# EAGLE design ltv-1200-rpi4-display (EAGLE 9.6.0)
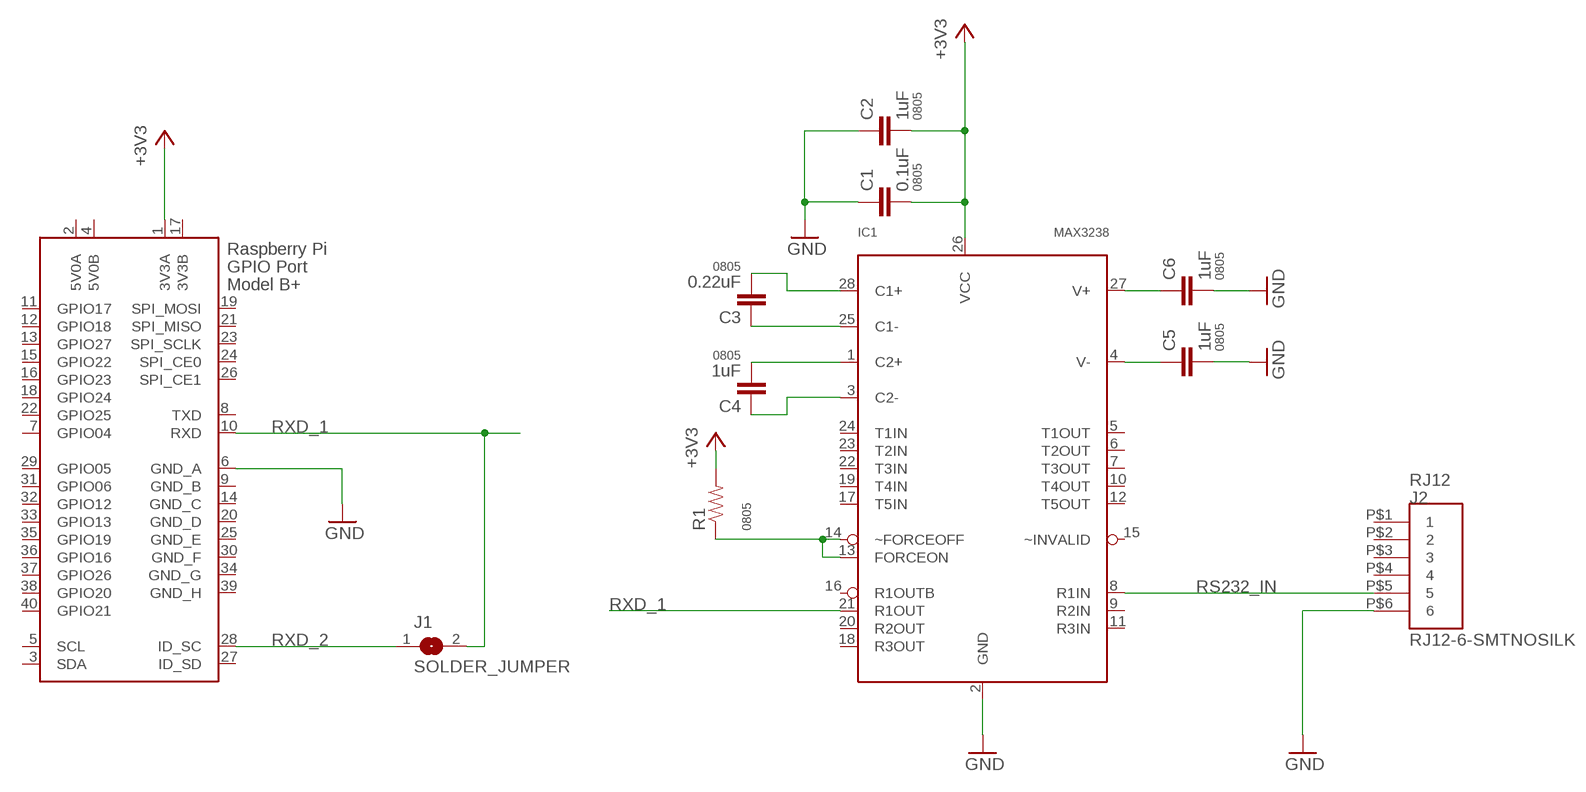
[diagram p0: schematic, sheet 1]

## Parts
C1  0.1uF  CAP0805  [0805]
C2  1uF  CAP0805  [0805]
C3  0.22uF  CAP0805  [0805]
C4  1uF  CAP0805  [0805]
C5  1uF  CAP0805  [0805]
C6  1uF  CAP0805  [0805]
IC1  MAX3238  [SSOP28]
J1  SOLDER_JUMPER  [SOLDER_JUMPER]
J2  RJ12-6-SMTNOSILK  [RJ12-6-SMT-NOSILK]
R1  RESISTOR0805-RES  [0805]
X1  RASPI_BOARD_B+#_F  [RASPI_BOARD_B+_FULL]

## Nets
+3V3: C1.2 C2.2 IC1.26(VCC) R1.2 X1.1(3V3A)
GND: C1.1 C2.1 C5.2 C6.2 IC1.2(GND) J2.P$6 X1.6(GND_A)
N$1: C3.2 IC1.28(C1+)
N$2: C3.1 IC1.25(C1-)
N$3: C4.2 IC1.1(C2+)
N$4: C4.1 IC1.3(C2-)
N$5: C6.1 IC1.27(V+)
N$6: C5.1 IC1.4(V-)
N$7: IC1.13(FORCEON) IC1.14(~FORCEOFF) R1.1
RS232_IN: IC1.8(R1IN) J2.P$5
RXD_1: IC1.21(R1OUT) J1.2 X1.10(RXD)
RXD_2: J1.1 X1.28(ID_SC)
Unconnected: IC1.5(T1OUT) IC1.6(T2OUT) IC1.7(T3OUT) IC1.9(R2IN) IC1.10(T4OUT) IC1.11(R3IN) IC1.12(T5OUT) IC1.15(~INVALID) IC1.16(R1OUTB) IC1.17(T5IN) IC1.18(R3OUT) IC1.19(T4IN) IC1.20(R2OUT) IC1.22(T3IN) IC1.23(T2IN) IC1.24(T1IN) J2.P$1 J2.P$2 J2.P$3 J2.P$4 X1.3(SDA) X1.5(SCL) X1.7(GPIO04) X1.8(TXD) X1.11(GPIO17) X1.12(GPIO18) X1.13(GPIO27) X1.15(GPIO22) X1.16(GPIO23) X1.18(GPIO24) X1.19(SPI_MOSI) X1.21(SPI_MISO) X1.22(GPIO25) X1.23(SPI_SCLK) X1.24(SPI_CE0) X1.26(SPI_CE1) X1.27(ID_SD) X1.29(GPIO05) X1.31(GPIO06) X1.32(GPIO12) X1.33(GPIO13) X1.35(GPIO19) X1.36(GPIO16) X1.37(GPIO26) X1.38(GPIO20) X1.40(GPIO21)

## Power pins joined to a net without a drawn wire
3V3B: X1.17(3V3B)
5V0A: X1.2(5V0A)
5V0B: X1.4(5V0B)
GND_B: X1.9(GND_B)
GND_C: X1.14(GND_C)
GND_D: X1.20(GND_D)
GND_E: X1.25(GND_E)
GND_F: X1.30(GND_F)
GND_G: X1.34(GND_G)
GND_H: X1.39(GND_H)

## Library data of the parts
C1-C6 = passives:CAP: Capacitor; PACKAGE: 0805
IC1 = comm:MAX3238: RS232 TRANSEIVER; AVAILABILITY: Unavailable; DESCRIPTION: 5/3 Transceiver Full RS232 28-SSOP; MF: Maxim Integrated; MP: MAX3238; PACKAGE: None; PRICE: None
J1 = connector:SOLDER_JUMPER
J2 = connector:RJ12-6-SMT
R1 = passives:RESISTOR: Resistor; PACKAGE: 0805
X1 = raspberrypi_bastelstube_v13:RASPI_BOARD_B+#: Raspberry Pi GPIO connector with markings for the outer dimensions of the Raspberry Pi board model B+ with different sets of drill holes or mounting pads All pins connected

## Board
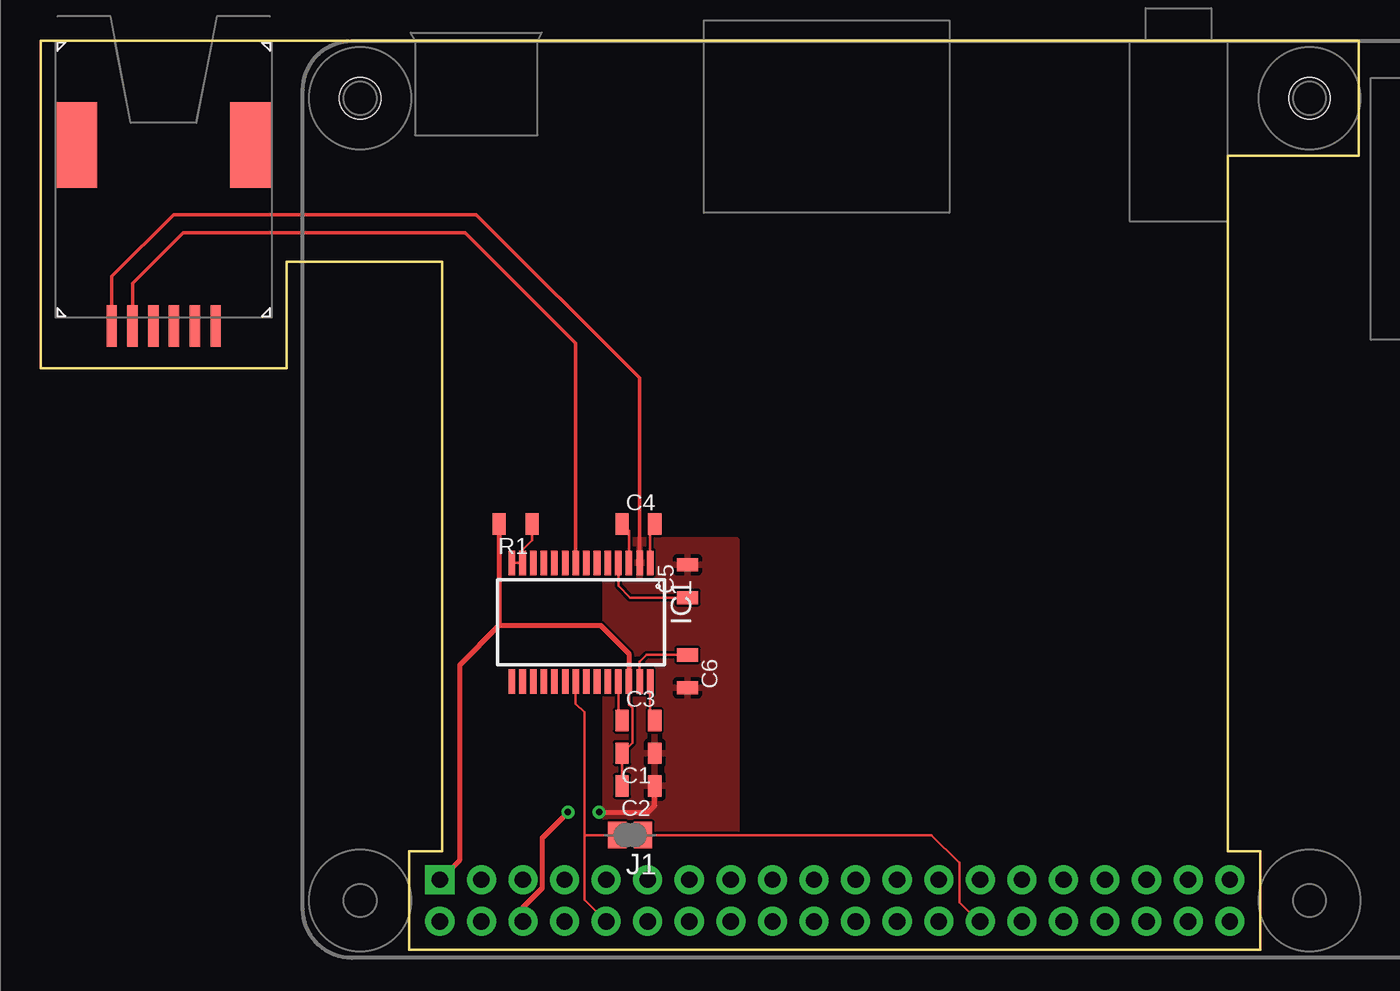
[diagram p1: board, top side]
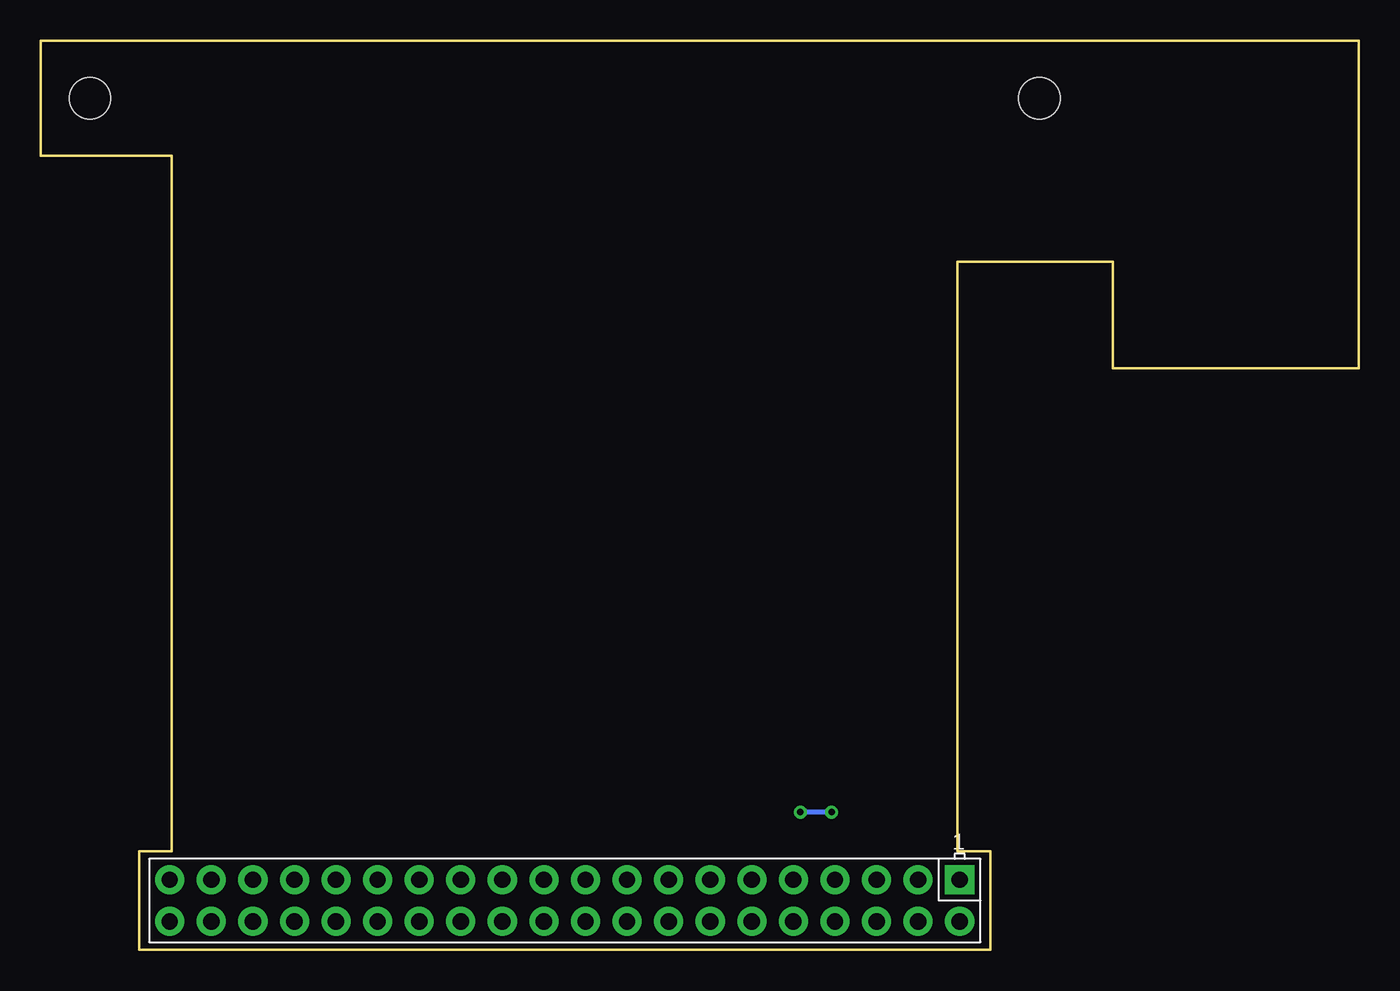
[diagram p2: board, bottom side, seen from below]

Size 80.5 x 55.5 mm. Coordinates in mm from the lower left corner, seen from the top.
Outline: 22.5,0 22.5,6 24.5,6 24.5,42 15,42 15,35.5 0,35.5 0,55.5 80.5,55.5 80.5,48.5 72.5,48.5 72.5,6 74.5,6 74.5,0 22.5,0
Copper layers (1*16): Top 0.035mm / dielectric 1.5mm / Bottom 0.035mm
Design rules "default *": minimum track width 6mil, minimum drill 0.35mm, track to track 6mil, track to pad 6mil, pad to pad 6mil, via to via 6mil, smd to smd 6mil, copper to edge 16mil, drill to drill 6mil, minimum pad ring 10mil, minimum via ring 8mil, stop-mask expansion 4mil, vias tented up to drill 0mil, thermal gap 10mil
Holes 2.5 mm at 19.5,52 77.5,52

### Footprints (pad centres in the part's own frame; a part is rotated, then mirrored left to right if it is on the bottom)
0805 = smd 0.8 x 1.3: 1 -1,0; 2 1,0
SSOP28 = smd 0.4 x 1.5: 1 -4.225,-3.625; 2 -3.575,-3.625; 3 -2.925,-3.625; 4 -2.275,-3.625; 5 -1.625,-3.625; 6 -0.975,-3.625; 7 -0.325,-3.625; 8 0.325,-3.625; 9 0.975,-3.625; 10 1.625,-3.625; 11 2.275,-3.625; 12 2.925,-3.625; 13 3.575,-3.625; 14 4.225,-3.625; 15 4.225,3.625; 16 3.575,3.625; 17 2.925,3.625; 18 2.275,3.625; 19 1.625,3.625; 20 0.975,3.625; 21 0.325,3.625; 22 -0.325,3.625; 23 -0.975,3.625; 24 -1.625,3.625; 25 -2.275,3.625; 26 -2.925,3.625; 27 -3.575,3.625; 28 -4.225,3.625
SOLDER_JUMPER = smd 1.118 x 1.6: 1 -0.787,0; 2 0.787,0
RJ12-6-SMT-NOSILK = smd 0.635 x 2.54: P$1 -3.175,17.399; P$2 -1.905,17.399; P$3 -0.635,17.399; P$4 0.635,17.399; P$5 1.905,17.399; P$6 3.175,17.399 | smd 2.54 x 5.207: P$7 -5.334,6.35; P$8 5.334,6.35
RASPI_BOARD_B+_FULL = drill 1 pad 1.778 square: 1 8.37,51.23 | drill 1 pad 1.778: 2 8.37,53.77; 3 10.91,51.23; 4 10.91,53.77; 5 13.45,51.23; 6 13.45,53.77; 7 15.99,51.23; 8 15.99,53.77; 9 18.53,51.23; 10 18.53,53.77; 11 21.07,51.23; 12 21.07,53.77; 13 23.61,51.23; 14 23.61,53.77; 15 26.15,51.23; 16 26.15,53.77; 17 28.69,51.23; 18 28.69,53.77; 19 31.23,51.23; 20 31.23,53.77; 21 33.77,51.23; 22 33.77,53.77; 23 36.31,51.23; 24 36.31,53.77; 25 38.85,51.23; 26 38.85,53.77; 27 41.39,51.23; 28 41.39,53.77; 29 43.93,51.23; 30 43.93,53.77; 31 46.47,51.23; 32 46.47,53.77; 33 49.01,51.23; 34 49.01,53.77; 35 51.55,51.23; 36 51.55,53.77; 37 54.09,51.23; 38 54.09,53.77; 39 56.63,51.23; 40 56.63,53.77

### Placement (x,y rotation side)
C1  36.5,12 180 top
C2  36.5,10 180 top
C3  36.5,14 0 top
C4  36.5,26 0 top
C5  39.5,22.5 90 top
C6  39.5,17 270 top
IC1  33,20 180 top
J1  36,7 180 top
J2  7.5,55.5 180 top
R1  29,26 180 top
U$1  [OSOYOO_DSI_5_TOUCHSCREEN]  19.5,3 0 top
X1  16,55.5 180 bottom

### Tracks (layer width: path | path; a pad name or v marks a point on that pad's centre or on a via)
+3V3
  Top 0.152: IC1.26 35.92,14.95 36.13,14.74 36.13,12.63 C1.2 C2.2
  Top 0.305: X1.1 25.6,5.5 25.6,17.4 28,19.8 28.1,19.8 | 28.1,19.8 34.2,19.8 35.92,18.07 IC1.26 | R1.2 28,19.9 28.1,19.8
GND  (via drill 0.4)
  Top 0.203: J2.P$6 4.32,41.12 8.1,44.9 26.6,44.9 36.58,34.92 IC1.2
  Top 0.305: X1.6 29.45,2.58 30.64,3.78 30.64,6.84 v32.2,8.4 | v34.1,8.4 37.1,8.4 37.5,8.8 C2.1
  Bottom 0.305: v32.2,8.4 v34.1,8.4
  pour Top: 34.5,25 42.5,25 42.5,7 34.5,7
N$1
  Top 0.152: IC1.28 37.23,14.28 C3.2
N$2
  Top 0.152: IC1.25 35.27,14.22 C3.1
N$3
  Top 0.152: IC1.1 37.23,25.73 C4.2
N$4
  Top 0.152: IC1.3 35.92,25.57 C4.1
N$5
  Top 0.152: IC1.27 36.58,17.57 37,18 C6.1
N$6
  Top 0.152: IC1.4 35.27,22.23 36,21.5 C5.1
N$7
  Top 0.152: IC1.14 IC1.13 29.43,24.43 30,25 R1.1
RS232_IN
  Top 0.203: J2.P$5 5.6,40.7 8.7,43.8 25.9,43.8 32.67,37.02 IC1.8
RXD_1
  Top 0.152: X1.10 33.2,3.06 33.2,7 | IC1.21 32.67,15.03 33.2,14.5 33.2,7 | J1.2 33.2,7
RXD_2
  Top 0.152: J1.1 54.4,7 56.1,5.3 56.1,2.9 57.27,1.73 X1.28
